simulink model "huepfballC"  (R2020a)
settings: Solver=ode45  StartTime=0.0  StopTime=50  RelTol=1e-3  EnableMultiTasking=on

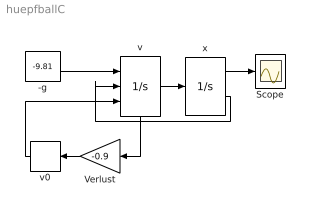
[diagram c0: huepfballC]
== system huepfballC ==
  -g : Constant  Value=-9.81
  Scope : Scope
  Verlust : Gain  Gain=-0.9  SaturateOnIntegerOverflow=on
  v : Integrator  ExternalReset=falling  InitialConditionSource=external  LowerSaturationLimit=0  ShowStatePort=on
  v0 : InitialCondition  Value=10
  x : Integrator  InitialCondition=20  LimitOutput=on  LowerSaturationLimit=0  ShowSaturationPort=on
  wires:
  v/1 -> x/1
  x/1 -> Scope/1
  -g/1 -> v/1
  x/2 -> v/2
  Verlust/1 -> v0/1
  v0/1 -> v/3
  v/State -> Verlust/1
